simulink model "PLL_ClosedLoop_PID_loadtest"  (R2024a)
settings: Solver=VariableStepAuto  StartTime=0.0  StopTime=1  MaxStep=1e-6  RelTol=1e-3
libraries: spsIGBTDiodeLib x6, spsThreePhaseSeriesRLCBranchLib x6, spsDiodeLib x6, spsGroundLib x4, spsThreePhaseBreakerLib x4, spsSeriesRLCBranchLib x3, spsThreePhaseVIMeasurementLib x3, spsMultimeterLib x3, spsThreePhaseSourceLib x2, spsTHDLib x2, spsPower3phInstantaneousLib x2, slpidlib x1

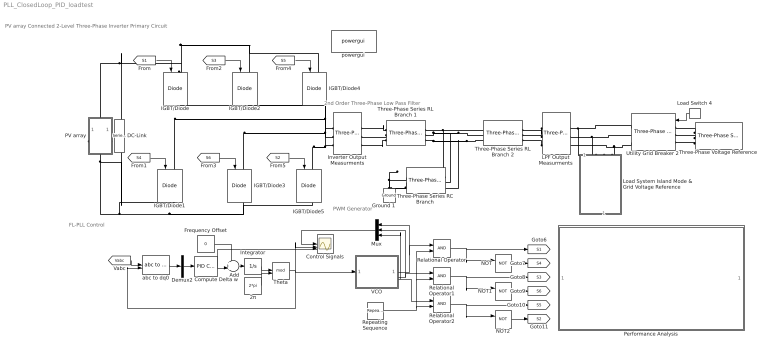
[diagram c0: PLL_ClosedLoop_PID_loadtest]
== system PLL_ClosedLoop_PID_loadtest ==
  note: FL-PLL Control
  note: PV array Connected 2-Level Three-Phase Inverter Primary Circuit
  note: PWM Generator
  note: 2nd Order Three-Phase Low Pass Filter
  2π : Constant  Value=2*pi  OutDataTypeStr=Inherit: Inherit via back propagation
  Add : Sum  Inputs=++|
  Compute Delta w : slpidlib/PID Controller  Controller=PID  Form=Parallel  TimeDomain=Continuous-time  UseExternalTs=off  SampleTime=-1  IntegratorMethod=Forward Euler  FilterMethod=Forward Euler  ControllerParametersSource=internal  P=0.00014180140811758  I=2.71241047007588e-05  UseKiTs=off  D=-2.98827242572439e-05  UseExternalDerivativeSource=off  N=1.72044274974478  UseFilter=on  TunerSelectOption=Transfer Function Based (PID Tuner App)  InitialConditionSource=internal  InitialConditionForIntegrator=0  InitialConditionForFilter=0  DifferentiatorICPrevScaledInput=0  ExternalReset=none  TrackingMode=off  Kt=1  LimitOutput=off  SatLimitsSource=internal  UpperSaturationLimit=inf  LowerSaturationLimit=-inf  LinearizeAsGain=on  AntiWindupMode=none  Kb=1  LimitIntegrator=off  UpperIntegratorSaturationLimit=inf  LowerIntegratorSaturationLimit=-inf  POutMin=[]  POutMax=[]  IOutMin=[]  IOutMax=[]  DOutMin=[]  DOutMax=[]  NOutMin=[]  NOutMax=[]  SumOutMin=[]  SumOutMax=[]  SaturationOutMin=[]  SaturationOutMax=[]  PParamMin=[]  PParamMax=[]  IParamMin=[]  IParamMax=[]  DParamMin=[]  DParamMax=[]  NParamMin=[]  NParamMax=[]  KbParamMin=[]  KbParamMax=[]  KtParamMin=[]  KtParamMax=[]  KbOutMin=[]  KbOutMax=[]  KtOutMin=[]  KtOutMax=[]  IntegratorOutMin=[]  IntegratorOutMax=[]  FilterOutMin=[]  FilterOutMax=[]  SumI1OutMin=[]  SumI1OutMax=[]  SumI2OutMin=[]  SumI2OutMax=[]  SumI3OutMin=[]  SumI3OutMax=[]  SumI4OutMin=[]  SumI4OutMax=[]  SumDOutMin=[]  SumDOutMax=[]  DifferentiatorOutMin=[]  DifferentiatorOutMax=[]  FilterDiffOutCoefMin=[]  FilterDiffOutCoefMax=[]  ReciprocalOutMin=[]  ReciprocalOutMax=[]  SumDenOutMin=[]  SumDenOutMax=[]  SumNumOutMin=[]  SumNumOutMax=[]  DivideOutMin=[]  DivideOutMax=[]  UdiffTsProdOutMin=[]  UdiffTsProdOutMax=[]  NTsProdOutMin=[]  NTsProdOutMax=[]  UintegralTsProdOutMin=[]  UintegralTsProdOutMax=[]  UngainTsProdOutMin=[]  UngainTsProdOutMax=[]  ClampingZeroOutDataTypeStr=Inherit: Inherit via back propagation  ClampingZeroOutMin=[]  ClampingZeroOutMax=[]  FilterDenConstantOutDataTypeStr=Inherit: Inherit via back propagation  FilterDenConstantOutMin=[]  FilterDenConstantOutMax=[]  PCopyOutDataTypeStr=Inherit: Inherit via back propagation  PCopyOutMin=[]  PCopyOutMax=[]  NCopyOutDataTypeStr=Inherit: Inherit via back propagation  NCopyOutMin=[]  NCopyOutMax=[]  IntegratorContinuousStateAttributes=''  IntegratorStateMustResolveToSignalObject=off  IntegratorRTWStateStorageClass=Auto  FilterContinuousStateAttributes=''  FilterStateMustResolveToSignalObject=off  FilterRTWStateStorageClass=Auto  ParallelPVariant=InternalParameters  IdealPVariant=Disabled  IVariant=InternalParameters  DVariant=InternalParameters  IntegratorVariant=Continuous  SatVariant=Disabled  AWVariant=Passthrough  PCopyVariant=Disabled  TRVariant=Disabled  FdbkBlocksVariant=Forward  IdealPFdbkVariant=Disabled  SatFdbkVariant=Disabled  DerivativeFilterVariant=ContFilter  NVariant=InternalParameters  NCopyVariant=Disabled  FilterICVariant=InternalICsFilter  IntegratorICVariant=InternalICs  ExternalResetVariant=Disabled  TRSumVariant=Passthrough  SumFdbkVariant=Disabled  SumVariant=Sum_PID  TsampFilterVariant=InternalTs  TsampNgainVariant=Passthrough  TsampIntegralVariant=Disabled_SignalSpec  ExternalSaturationOutDataTypeStr=Inherit: Same as second input  DerivativeSourceVariant=ErrorSignal
  Control Signals : Scope  NumInputPorts=3
  DC-Link : spsSeriesRLCBranchLib/Series RLC Branch  LConnTagsString=__new0  RConnTagsString=__new0  BranchType=RC  Resistance=20e-3  Inductance=1e-3  SetiL0=off  InitialCurrent=0  Capacitance=81e-6  Setx0=off  InitialVoltage=0  Measurements=None
  Demux2 : Demux  Outputs=3
  Frequency Offset : Constant  Value=0
  Ground 1 : spsGroundLib/Ground  LConnTagsString=a
  IGBT/Diode{,1..5} (6 alike) : spsIGBTDiodeLib/IGBT//Diode  Ron=1e-3  Rs=1e5  Cs=inf  Measurements=off
  Integrator : Integrator
  Inverter Output Measurments : spsThreePhaseVIMeasurementLib/Three-Phase V-I Measurement  VoltageMeasurement=phase-to-phase  SetLabelV=on  LabelV=Vinv  Vpu=off  VpuLL=off  CurrentMeasurement=yes  SetLabelI=on  LabelI=Iinv  Ipu=off  Pbase=100e6  Vbase=500e3  OutputType=Complex  PhasorSimulation=off  PSBequivalent=0
  LPF Output Measurments : spsThreePhaseVIMeasurementLib/Three-Phase V-I Measurement  VoltageMeasurement=phase-to-phase  SetLabelV=on  LabelV=Vabc  Vpu=off  VpuLL=off  CurrentMeasurement=yes  SetLabelI=on  LabelI=Iabc  Ipu=off  Pbase=100e6  Vbase=500e3  OutputType=Complex  PhasorSimulation=off  PSBequivalent=0
  Load Switch 4 : DiscretePulseGenerator  PulseType=Time based  Period=1.2  PulseWidth=50  PhaseDelay=0.6
  Load System Island Mode & Grid Voltage Reference : Subsystem
  Mux : Mux  Inputs=3
  NOT : Logic  Operator=NOT  IconShape=distinctive  AllPortsSameDT=off  OutDataTypeStr=boolean
  NOT1 : Logic  Operator=NOT  IconShape=distinctive  AllPortsSameDT=off  OutDataTypeStr=boolean
  NOT2 : Logic  Operator=NOT  IconShape=distinctive  AllPortsSameDT=off  OutDataTypeStr=boolean
  PV array : Subsystem
  Performance Analysis : Subsystem
  Relational Operator : RelationalOperator  OutDataTypeStr=boolean  RndMeth=Simplest
  Relational Operator1 : RelationalOperator  OutDataTypeStr=boolean  RndMeth=Simplest
  Relational Operator2 : RelationalOperator  OutDataTypeStr=boolean  RndMeth=Simplest
  Repeating Sequence : simulink/Sources/Repeating Sequence  rep_seq_t=[0 1 2 3]/30000  rep_seq_y=[0 1 -1 0]
  Theta : Math  Operator=mod
  Three-Phase Series RC Branch : spsThreePhaseSeriesRLCBranchLib/Three-Phase Series RLC Branch  LConnTagsString=A|B|C  RConnTagsString=A|B|C  BranchType=RC  Resistance=20e-3  Inductance=500e-4  Capacitance=81e-6  Measurements=None
  Three-Phase Series RL Branch 1 : spsThreePhaseSeriesRLCBranchLib/Three-Phase Series RLC Branch  LConnTagsString=A|B|C  RConnTagsString=A|B|C  BranchType=RL  Resistance=20e-3  Inductance=45e-6  Capacitance=1e-6  Measurements=None
  Three-Phase Series RL Branch 2 : spsThreePhaseSeriesRLCBranchLib/Three-Phase Series RLC Branch  LConnTagsString=A|B|C  RConnTagsString=A|B|C  BranchType=RL  Resistance=20e-3  Inductance=45e-6  Capacitance=1e-6  Measurements=None
  Three-Phase Voltage Reference : spsThreePhaseSourceLib/Three-Phase Source  InternalConnection=Yg  VoltagePhases=off  Voltage=240  PhaseAngle=61.4  Voltage_phases=[25e3 25e3 25e3]/sqrt(3)  PhaseAngles_phases=[0 -120 +120]  Frequency=50  NonIdealSource=on  SpecifyImpedance=off  Resistance=0.8929  Inductance=16.58e-3  ShortCircuitLevel=100e6  BaseVoltage=240  XRratio=7  BusType=swing  Pref=10e3  Qref=0  Prefabc=[10e3, 10e3, 10e3]  Qrefabc=[0, 0, 0]  Qmin=-inf  Qmax=inf
  Utility Grid Breaker 2 : spsThreePhaseBreakerLib/Three-Phase Breaker  InitialState=open  SwitchA=on  SwitchB=on  SwitchC=on  SwitchTimes="[1/60  5/60]"  External=on  BreakerResistance=0.01  SnubberResistance=1e6  SnubberCapacitance=inf  Measurements=None
  VCO : Subsystem
  abc to dq0 : spsabctodq0Lib/abc to dq0  Alignment=90 degrees behind phase A axis
  powergui : spspowerguiLib/powergui  Priority=1  SimulationMode=Discrete  SampleTime=1e-6  frequency=50  Iterations=50  frequencyindice=0  Pbase=100e6  ErrMax=1e-4  UnitsV=kV  UnitsW=MW  buscounter=0  FunctionMessages=off  echomessages=off  EnableUseOfTLC=off  CurrentSourceSwitches=off  DisableSnubberDevices=off  DisableRonSwitches=off  DisableVfSwitches=off  DisplayEquations=off  AutomaticDiscreteSolvers=off  SolverType=Tustin/Backward Euler (TBE)  Interpol=off  ExternalGateDelay=off  methode=off  Ts=100  x0status=blocks  SPID=on  SwTol=0  HookPort=off  NonlinearTolerance=1e-4  nMaxIteration=100  ContinueOnMaxIteration=off  RestoreLinks=warning  ResistiveCurrentMeasurement=off  Frange=[0:2:500]  Ylog=off  Xlog=on  ShowGrid=off  save=off  variable=ZData  structure=0  ZoomFFT=off  StartTime=0.0  cycles=1  DisplayStyle=1  fundamental=60  FreqAxis=off  MaxFrequency=1000  frequencyindicesteady=1  RmsSteady=1  display=off
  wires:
  [S3] -> IGBT/Diode2/1
  [S6] -> IGBT/Diode3/1
  [S2] -> IGBT/Diode5/1
  [S4] -> IGBT/Diode1/1
  [S1] -> IGBT/Diode/1
  [S5] -> IGBT/Diode4/1
  Demux2/2 -> Compute Delta w/1
  2π/1 -> Theta/2
  Integrator/1 -> Theta/1
  Theta/1 -> abc to dq0/2, VCO/1(Theta), Control Signals/2
  Frequency Offset/1 -> Add/1
  Compute Delta w/1 -> Control Signals/3, Add/2
  Add/1 -> Integrator/1
  NOT2/1 -> [S2]
  NOT/1 -> [S4]
  Relational Operator2/1 -> [S5], NOT2/1
  Repeating Sequence/1 -> Relational Operator2/2, Relational Operator1/2, Relational Operator/2
  NOT1/1 -> [S6]
  Relational Operator1/1 -> [S3], NOT1/1
  VCO/3(Vref C) -> Mux/3, Relational Operator2/1
  Relational Operator/1 -> [S1], NOT/1
  VCO/2(Vref B) -> Mux/2, Relational Operator1/1
  [Vabc] -> abc to dq0/1
  Load Switch 4/1 -> Utility Grid Breaker 2/1
  Mux/1 -> Control Signals/1
  VCO/1(Vref A) -> Mux/1, Relational Operator/1
  abc to dq0/1 -> Demux2/1
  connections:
  IGBT/Diode/LConn1 -- IGBT/Diode2/LConn1 -- IGBT/Diode4/LConn1 -- DC-Link/LConn1 -- PV array/LConn1
  Inverter Output Measurments/LConn1 -- IGBT/Diode1/LConn1 -- IGBT/Diode/RConn1
  Inverter Output Measurments/LConn2 -- IGBT/Diode3/LConn1 -- IGBT/Diode2/RConn1
  LPF Output Measurments/RConn1 -- Utility Grid Breaker 2/RConn1 -- Load System Island Mode & Grid Voltage Reference/LConn1
  LPF Output Measurments/RConn2 -- Utility Grid Breaker 2/RConn2 -- Load System Island Mode & Grid Voltage Reference/LConn2
  Inverter Output Measurments/LConn3 -- IGBT/Diode5/LConn1 -- IGBT/Diode4/RConn1
  Load System Island Mode & Grid Voltage Reference/LConn3 -- LPF Output Measurments/RConn3 -- Utility Grid Breaker 2/RConn3
  PV array/RConn1 -- IGBT/Diode5/RConn1 -- IGBT/Diode3/RConn1 -- IGBT/Diode1/RConn1 -- DC-Link/RConn1
  LPF Output Measurments/LConn2 -- Three-Phase Series RL Branch 2/RConn2
  Three-Phase Series RL Branch 1/LConn1 -- Inverter Output Measurments/RConn1
  LPF Output Measurments/LConn3 -- Three-Phase Series RL Branch 2/RConn3
  Three-Phase Series RL Branch 1/LConn2 -- Inverter Output Measurments/RConn2
  LPF Output Measurments/LConn1 -- Three-Phase Series RL Branch 2/RConn1
  Three-Phase Series RL Branch 1/LConn3 -- Inverter Output Measurments/RConn3
  Three-Phase Series RL Branch 1/RConn3 -- Three-Phase Series RL Branch 2/LConn3 -- Three-Phase Series RC Branch/LConn3
  Three-Phase Series RC Branch/LConn1 -- Three-Phase Series RL Branch 2/LConn1 -- Three-Phase Series RL Branch 1/RConn1
  Ground 1/LConn1 -- Three-Phase Series RC Branch/RConn3 -- Three-Phase Series RC Branch/RConn2 -- Three-Phase Series RC Branch/RConn1
  Three-Phase Series RL Branch 1/RConn2 -- Three-Phase Series RL Branch 2/LConn2 -- Three-Phase Series RC Branch/LConn2
  Three-Phase Voltage Reference/RConn1 -- Utility Grid Breaker 2/LConn1
  Three-Phase Voltage Reference/RConn2 -- Utility Grid Breaker 2/LConn2
  Three-Phase Voltage Reference/RConn3 -- Utility Grid Breaker 2/LConn3

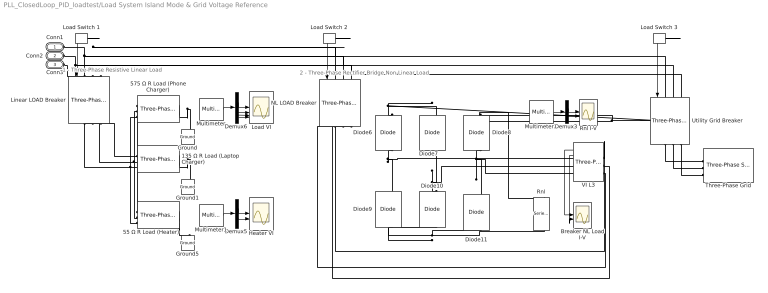
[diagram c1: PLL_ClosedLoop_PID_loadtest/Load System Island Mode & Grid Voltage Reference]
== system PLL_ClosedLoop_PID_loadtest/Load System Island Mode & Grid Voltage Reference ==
  note: 1 - Three-Phase Resistive Linear Load
  note: 2 - Three-Phase Rectifier Bridge Non-Linear Load
  135 Ω R Load (Laptop Charger) : spsThreePhaseSeriesRLCBranchLib/Three-Phase Series RLC Branch  LConnTagsString=A|B|C  RConnTagsString=A|B|C  BranchType=R  Resistance=135  Inductance=5.1e-3  Capacitance=1e-6  Measurements=Branch voltages and currents
  55 Ω R Load (Heater) : spsThreePhaseSeriesRLCBranchLib/Three-Phase Series RLC Branch  LConnTagsString=A|B|C  RConnTagsString=A|B|C  BranchType=R  Resistance=55  Inductance=5.1e-3  Capacitance=1e-6  Measurements=Branch voltages and currents
  575 Ω R Load (Phone Charger) : spsThreePhaseSeriesRLCBranchLib/Three-Phase Series RLC Branch  LConnTagsString=A|B|C  RConnTagsString=A|B|C  BranchType=R  Resistance=575  Inductance=5.1e-3  Capacitance=1e-6  Measurements=Branch voltages and currents
  Breaker NL Load I-V : Scope  NumInputPorts=2
  Demux3 : Demux  Outputs=2
  Demux5 : Demux  Outputs=2
  Demux6 : Demux
  Diode{6..11} (6 alike) : spsDiodeLib/Diode  Ron=0.001  Lon=0  Vf=0.8  IC=0  UseSnubber=0  Rs=10e+6  Cs=250e-9  Measurements=off
  Ground : spsGroundLib/Ground  LConnTagsString=a
  Ground1 : spsGroundLib/Ground  LConnTagsString=a
  Ground5 : spsGroundLib/Ground  LConnTagsString=a
  Heater VI : Scope  NumInputPorts=2
  Linear LOAD Breaker : spsThreePhaseBreakerLib/Three-Phase Breaker  InitialState=open  SwitchA=on  SwitchB=on  SwitchC=on  SwitchTimes="[1/60  5/60]"  External=on  BreakerResistance=0.01  SnubberResistance=1e6  SnubberCapacitance=inf  Measurements=None
  Load Switch 1 : DiscretePulseGenerator  PulseType=Time based  Period=0.6  PulseWidth=100/3
  Load Switch 2 : DiscretePulseGenerator  PulseType=Time based  Period=0.6  PulseWidth=100/3  PhaseDelay=0.2
  Load Switch 3 : DiscretePulseGenerator  PulseType=Time based  Period=0.6  PulseWidth=100/3  PhaseDelay=0.4
  Load VI : Scope  NumInputPorts=4
  Multimeter : spsMultimeterLib/Multimeter  L=20  sel=[8 2 18 12]  yselected={}  Gain=[1 1 1 1]  OutputType=Complex  PlotAtSimulationStop=off  PhasorSimulation=off
  Multimeter1 : spsMultimeterLib/Multimeter  L=20  sel=[5 15]  yselected={}  Gain=[1 1]  OutputType=Complex  PlotAtSimulationStop=off  PhasorSimulation=off
  Multimeter2 : spsMultimeterLib/Multimeter  L=20  sel=[1 11]  yselected={}  Gain=[1 1]  OutputType=Complex  PlotAtSimulationStop=off  PhasorSimulation=off
  NL LOAD Breaker : spsThreePhaseBreakerLib/Three-Phase Breaker  InitialState=open  SwitchA=on  SwitchB=on  SwitchC=on  SwitchTimes="[1/60  5/60]"  External=on  BreakerResistance=0.01  SnubberResistance=1e6  SnubberCapacitance=inf  Measurements=None
  Rnl : spsSeriesRLCBranchLib/Series RLC Branch  LConnTagsString=__new0  RConnTagsString=__new0  BranchType=R  Resistance=60  Inductance=1e-6  SetiL0=off  InitialCurrent=0  Capacitance=0.01598  Setx0=off  InitialVoltage=0  Measurements=Branch voltage and current
  Rnl I-V : Scope  NumInputPorts=2
  Three-Phase Grid : spsThreePhaseSourceLib/Three-Phase Source  InternalConnection=Yg  VoltagePhases=off  Voltage=240  PhaseAngle=0  Voltage_phases=[25e3 25e3 25e3]/sqrt(3)  PhaseAngles_phases=[0 -120 +120]  Frequency=50  NonIdealSource=on  SpecifyImpedance=off  Resistance=0.8929  Inductance=16.58e-3  ShortCircuitLevel=100e6  BaseVoltage=240  XRratio=7  BusType=swing  Pref=10e3  Qref=0  Prefabc=[10e3, 10e3, 10e3]  Qrefabc=[0, 0, 0]  Qmin=-inf  Qmax=inf
  Utility Grid Breaker : spsThreePhaseBreakerLib/Three-Phase Breaker  InitialState=open  SwitchA=on  SwitchB=on  SwitchC=on  SwitchTimes="[1/60  5/60]"  External=on  BreakerResistance=0.01  SnubberResistance=1e6  SnubberCapacitance=inf  Measurements=None
  VI L3 : spsThreePhaseVIMeasurementLib/Three-Phase V-I Measurement  VoltageMeasurement=phase-to-phase  SetLabelV=off  LabelV=Vabc  Vpu=off  VpuLL=off  CurrentMeasurement=yes  SetLabelI=off  LabelI=Iabc  Ipu=off  Pbase=100e6  Vbase=500e3  OutputType=Complex  PhasorSimulation=off  PSBequivalent=0
  Conn1 : PMIOPort  Side=Left
  Conn2 : PMIOPort  Port=2  Side=Left
  Conn3 : PMIOPort  Port=3  Side=Left
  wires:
  Demux5/2 -> Heater VI/2
  Demux6/2 -> Load VI/2
  Demux6/4 -> Load VI/4
  Demux6/1 -> Load VI/1
  Multimeter/1 -> Demux6/1
  Demux6/3 -> Load VI/3
  Demux5/1 -> Heater VI/1
  Multimeter1/1 -> Demux5/1
  Load Switch 1/1 -> Linear LOAD Breaker/1
  Load Switch 2/1 -> NL LOAD Breaker/1
  Load Switch 3/1 -> Utility Grid Breaker/1
  Multimeter2/1 -> Demux3/1
  Demux3/1 -> Rnl I-V/1
  Demux3/2 -> Rnl I-V/2
  VI L3/2 -> Breaker NL Load I-V/2
  VI L3/1 -> Breaker NL Load I-V/1
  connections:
  55 Ω R Load (Heater)/LConn2 -- 135 Ω R Load (Laptop Charger)/LConn2 -- Linear LOAD Breaker/RConn2 -- 575 Ω R Load (Phone Charger)/LConn2
  55 Ω R Load (Heater)/LConn3 -- 135 Ω R Load (Laptop Charger)/LConn3 -- Linear LOAD Breaker/RConn3 -- 575 Ω R Load (Phone Charger)/LConn3
  55 Ω R Load (Heater)/RConn1 -- 55 Ω R Load (Heater)/RConn2 -- 55 Ω R Load (Heater)/RConn3 -- Ground5/LConn1
  55 Ω R Load (Heater)/LConn1 -- 135 Ω R Load (Laptop Charger)/LConn1 -- Linear LOAD Breaker/RConn1 -- 575 Ω R Load (Phone Charger)/LConn1
  575 Ω R Load (Phone Charger)/RConn1 -- Ground/LConn1 -- 575 Ω R Load (Phone Charger)/RConn3 -- 575 Ω R Load (Phone Charger)/RConn2
  135 Ω R Load (Laptop Charger)/RConn1 -- Ground1/LConn1 -- 135 Ω R Load (Laptop Charger)/RConn3 -- 135 Ω R Load (Laptop Charger)/RConn2
  Utility Grid Breaker/RConn1 -- Three-Phase Grid/RConn1
  Utility Grid Breaker/RConn3 -- Three-Phase Grid/RConn3
  Utility Grid Breaker/RConn2 -- Three-Phase Grid/RConn2
  Conn1/RConn1 -- NL LOAD Breaker/LConn1 -- Utility Grid Breaker/LConn1 -- Linear LOAD Breaker/LConn1
  Conn2/RConn1 -- NL LOAD Breaker/LConn2 -- Utility Grid Breaker/LConn2 -- Linear LOAD Breaker/LConn2
  Conn3/RConn1 -- NL LOAD Breaker/LConn3 -- Utility Grid Breaker/LConn3 -- Linear LOAD Breaker/LConn3
  Diode6/RConn1 -- Rnl/LConn1 -- Diode8/RConn1 -- Diode7/RConn1
  Diode6/LConn1 -- Diode9/RConn1 -- VI L3/RConn1
  Diode8/LConn1 -- Diode11/RConn1 -- VI L3/RConn3
  Diode9/LConn1 -- Rnl/RConn1 -- Diode11/LConn1 -- Diode10/LConn1
  Diode10/RConn1 -- Diode7/LConn1 -- VI L3/RConn2
  NL LOAD Breaker/RConn1 -- VI L3/LConn1
  VI L3/LConn2 -- NL LOAD Breaker/RConn2
  VI L3/LConn3 -- NL LOAD Breaker/RConn3

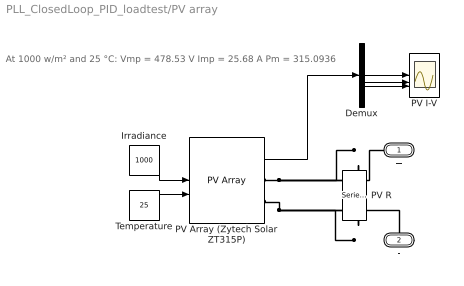
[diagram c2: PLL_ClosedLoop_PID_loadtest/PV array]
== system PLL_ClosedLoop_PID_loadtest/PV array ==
  note: At 1000 w/m² and 25 °C: Vmp = 478.53 V Imp = 25.68 A Pm = 315.0936
  Demux : Demux  Outputs=5
  Irradiance : Constant  Value=1000
  PV I-V : Scope  NumInputPorts=5
  PV Array (Zytech Solar ZT315P) : spsPVArrayLib/PV Array  Npar=3  Nser=13  PlotType=array @ 25 deg.C & specified irradiances  S_vec="[ 1000  500  100 ]"  Temp_C_vec="[ 45 25  ]"  ModuleName=Zytech Solar ZT315P  PlotWhenSelected=off  Pm=315.0936  Ncell=72  Voc=46.44  Isc=9.01  Vm=36.81  Im=8.56  beta_Voc_pc=-0.3199  alpha_Isc_pc=0.048302  beta_Voc=-0.14856  alpha_Isc=0.004352  IL=9.0792  I0=6.901e-11  nI=0.9809  Rsh=572.7811  Rs=0.50125  RobustModel=off  RobustCellTemperature=313.3991  BAL=on  Tc=1e-6  Tfilter=5e-5
  PV R : spsSeriesRLCBranchLib/Series RLC Branch  LConnTagsString=__new0  RConnTagsString=__new0  BranchType=R  Resistance=18.6  Inductance=1e-3  SetiL0=off  InitialCurrent=0  Capacitance=1e-6  Setx0=off  InitialVoltage=0  Measurements=None
  Temperature : Constant  Value=25
  + : PMIOPort  Side=Left
  - : PMIOPort  Port=2  Side=Right
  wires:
  PV Array (Zytech Solar ZT315P)/1 -> Demux/1
  Demux/3 -> PV I-V/3
  Temperature/1 -> PV Array (Zytech Solar ZT315P)/2
  Demux/2 -> PV I-V/2
  Irradiance/1 -> PV Array (Zytech Solar ZT315P)/1
  Demux/1 -> PV I-V/1
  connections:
  PV Array (Zytech Solar ZT315P)/RConn1 -- PV R/LConn1 -- +/RConn1
  PV Array (Zytech Solar ZT315P)/RConn2 -- PV R/RConn1 -- -/RConn1

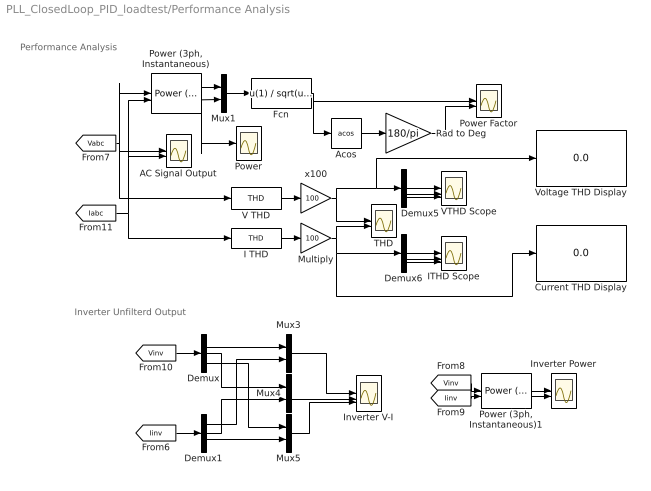
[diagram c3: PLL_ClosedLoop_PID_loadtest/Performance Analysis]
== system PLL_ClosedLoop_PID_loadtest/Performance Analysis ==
  note: Inverter Unfilterd Output
  note: Performance Analysis
  AC Signal Output : Scope  NumInputPorts=2
  Acos : Trigonometry  Operator=acos
  Current THD Display : Display
  Demux{,1,5..6} (4 alike) : Demux  Outputs=3
  Fcn : Fcn  Expr=u(1) / sqrt(u(1)^2 + u(2)^2)
  I THD : spsTHDLib/THD  Freq=50  Ts=0
  ITHD Scope : Scope  NumInputPorts=3
  Inverter V-I : Scope  NumInputPorts=3
  Inverter Power : Scope  NumInputPorts=2
  Multiply : Gain  Gain=100
  Mux{1,3..5} (4 alike) : Mux  Inputs=2
  Power : Scope
  "Power (3ph, Instantaneous)" : spsPower3phInstantaneousLib/Power (3ph, Instantaneous)
  "Power (3ph, Instantaneous)1" : spsPower3phInstantaneousLib/Power (3ph, Instantaneous)
  Power Factor : Scope  NumInputPorts=2
  Rad to Deg : Gain  Gain=180/pi
  THD : Scope  NumInputPorts=2
  V THD : spsTHDLib/THD  Freq=50  Ts=0
  VTHD Scope : Scope  NumInputPorts=3
  Voltage THD Display : Display
  x100 : Gain  Gain=100
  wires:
  x100/1 -> THD/1, Voltage THD Display/1, Demux5/1
  Fcn/1 -> Power Factor/1, Acos/1
  Demux5/2 -> VTHD Scope/2
  [Iabc] -> I THD/1, "Power (3ph, Instantaneous)"/2, AC Signal Output/2
  Demux6/3 -> ITHD Scope/3
  "Power (3ph, Instantaneous)"/1 -> Power/1, Mux1/1
  Demux6/2 -> ITHD Scope/2
  Multiply/1 -> Current THD Display/1, Demux6/1, THD/2
  Demux5/1 -> VTHD Scope/1
  Rad to Deg/1 -> Power Factor/2
  V THD/1 -> x100/1
  I THD/1 -> Multiply/1
  Demux5/3 -> VTHD Scope/3
  [Vabc] -> V THD/1, AC Signal Output/1, "Power (3ph, Instantaneous)"/1
  "Power (3ph, Instantaneous)"/2 -> Mux1/2
  Acos/1 -> Rad to Deg/1
  Mux1/1 -> Fcn/1
  Demux6/1 -> ITHD Scope/1
  "Power (3ph, Instantaneous)1"/1 -> Inverter Power/1
  "Power (3ph, Instantaneous)1"/2 -> Inverter Power/2
  [Iinv] -> "Power (3ph, Instantaneous)1"/2
  [Vinv] -> "Power (3ph, Instantaneous)1"/1
  Mux3/1 -> Inverter V-I/1
  Mux4/1 -> Inverter V-I/2
  Demux1/3 -> Mux5/2
  Demux1/1 -> Mux3/2
  [Vinv] -> Demux/1
  Demux/3 -> Mux5/1
  Demux/1 -> Mux3/1
  Demux1/2 -> Mux4/2
  Demux/2 -> Mux4/1
  Mux5/1 -> Inverter V-I/3
  [Iinv] -> Demux1/1

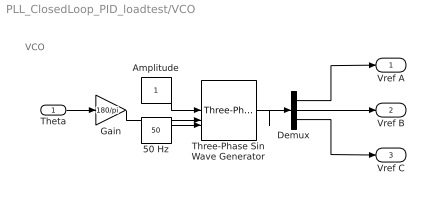
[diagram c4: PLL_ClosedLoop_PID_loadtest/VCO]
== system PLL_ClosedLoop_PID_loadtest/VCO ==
  note: VCO
  Theta : Inport
  50 Hz : Constant  Value=50  VectorParams1D=off  SampleTime=-1
  Amplitude : Constant  VectorParams1D=off  SampleTime=-1
  Demux : Demux  Outputs=3
  Gain : Gain  Gain=180/pi
  Three-Phase Sin Wave Generator : spsThreePhaseSineGeneratorLib/Three-Phase Sine Generator  Ts=0
  Vref A : Outport
  Vref B : Outport  Port=2
  Vref C : Outport  Port=3
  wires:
  50 Hz/1 -> Three-Phase Sin Wave Generator/3
  Amplitude/1 -> Three-Phase Sin Wave Generator/1
  Three-Phase Sin Wave Generator/1 -> Demux/1
  Demux/1 -> Vref A/1
  Demux/2 -> Vref B/1
  Demux/3 -> Vref C/1
  Theta/1 -> Gain/1
  Gain/1 -> Three-Phase Sin Wave Generator/2
